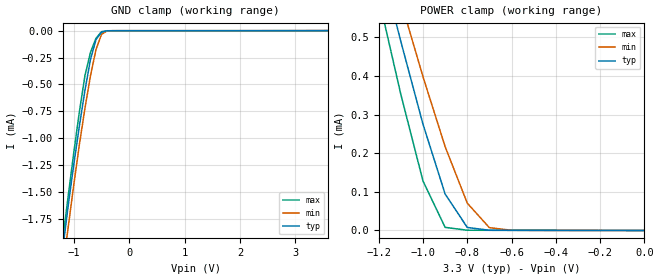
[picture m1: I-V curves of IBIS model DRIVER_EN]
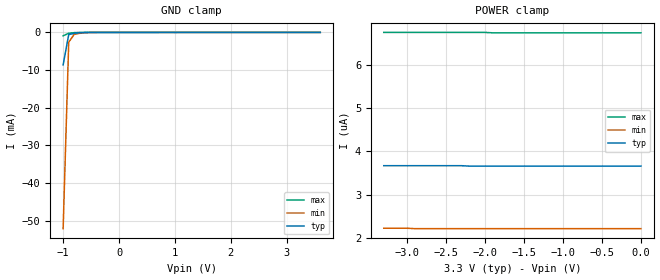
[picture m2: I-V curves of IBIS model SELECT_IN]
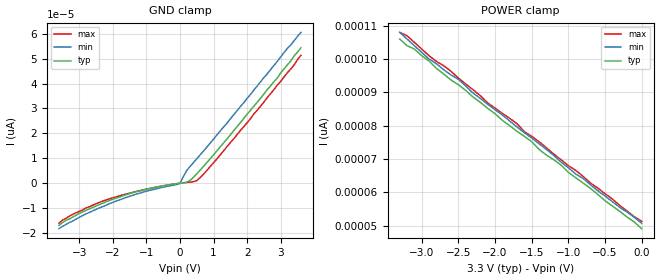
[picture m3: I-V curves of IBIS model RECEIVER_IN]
|   Texas Instruments Incorporated
|   Data Transmissions Products
|   IBIS Model for SN65LVDS125A
|   38DBT TSSOP Package
[IBIS Ver]   3.2
[Comment char]   |_char
[File name]   lvds125a.ibs
[File Rev]   2.1
[Date]   28Jan04
[Source]   File originated at Texas Instruments Incorporated.
   Data Transmission Products Group. All data based on
   Simulation Measurements.
[Notes]   Correlated to Silicon.
[Disclaimer]
(C) Copyright Texas Instruments Incorporated 2004
   All rights reserved
  Texas Instruments Incorporated hereby grants the user of this IBIS
model a non-exclusive, nontransferable license to use this IBIS model
under the following terms.  Before using this IBIS model, the user
should read this license.  If the user does not accept these terms,
the IBIS model should be returned to Texas Instruments within 30 days.
  The user is granted this license only to use the IBIS model and
is not granted rights to sell, load, rent, lease or license the IBIS
model in whole or in part, or in modified form to anyone other than
user.  User may modify the IBIS model to suit its specific applications
but rights to derivative works and such modifications shall belong to
Texas Instruments.
  This IBIS model is provided on an "AS IS" basis and Texas Instruments
makes absolutely no warranty with respect to the information contained
herein.  TEXAS INSTRUMENTS DISCLAIMS AND CUSTOMER WAIVES ALL WARRANTIES,
EXPRESS OR IMPLIED, INCLUDING WARRANTIES OF MERCHANTABILITY OR FITNESS
FOR A PARTICULAR PURPOSE. The entire risk as to quality and performance
is with the Customer. ACCORDINGLY, IN NO EVENT SHALL THE COMPANY BE LIABLE
FOR ANY DAMAGES, WHETHER IN CONTRACT OR TORT,INCLUDING ANY LOST PROFITS
OR OTHER INCIDENTAL, CONSEQUENTIAL, EXEMPLARY, OR PUNITIVE DAMAGES ARISING
OUT OF THE USE OR APPLICATION OF THE IBIS model provided in this package.
Further, Texas Instruments reserves the right to discontinue or make changes
without notice to any product herein to improve reliability, function, or
design. Texas Instruments does not convey any license under patent rights
or any other intellectual property rights, including those of third parties.
Contact Texas Instruments at ATTN:DATA TRANSMISSIONS
[Copyright]   Copyright 2004, Texas Instruments, All Rights Reserved
[Component]   SN65LVDS125A
[Manufacturer]  Texas Instruments Incorporated
[Package]
|   typ   min   max
R_pkg   0.045   0.036   0.057
L_pkg   2.694nH   2.290nH   3.177nH
C_pkg   0.156pF   0.076pF   0.259pF
[Pin]   signal_name   model_name   R_pin   L_pin   C_pin
1   S10   SELECT_IN   0.036   3.045nH   0.259pF
2   S11   SELECT_IN   0.051   3.013nH   0.189pF
3   1A   RECEIVER_IN   0.044   2.695nH   0.164pF
4   1B   RECEIVER_IN   0.047   2.362nH   0.079pF
5   S20   SELECT_IN   0.047   2.333nH   0.086pF
6   S21   SELECT_IN   0.047   2.298nH   0.085pF
7   2A   RECEIVER_IN   0.047   2.351nH   0.079pF
8   2B   RECEIVER_IN   0.044   2.706nH   0.165pF
9   GND   GND   0.049   2.999nH   0.188pF
10   VCC   POWER   0.039   3.039nH   0.257pF
11   GND   GND   0.038   3.044nH   0.258pF
12   3A   RECEIVER_IN   0.057   3.177nH   0.199pF
13   3B   RECEIVER_IN   0.044   2.825nH   0.173pF
14   S30   SELECT_IN   0.047   2.429nH   0.083pF
15   S31   SELECT_IN   0.049   2.383nH   0.090pF
16   4A   RECEIVER_IN   0.049   2.347nH   0.089pF
17   4B   RECEIVER_IN   0.047   2.290nH   0.076pF
18   S40   SELECT_IN   0.045   2.613nH   0.158pF
19   S41   SELECT_IN   0.044   2.883nH   0.181pF
20   VCC   POWER   0.039   3.044nH   0.256pF
21   GND   GND   0.038   3.044nH   0.258pF
22   4DE   DRIVER_EN   0.044   2.883nH   0.181pF
23   4Z   DRIVER_OUT   0.044   2.883nH   0.181pF
24   4Y   DRIVER_OUT   0.044   2.883nH   0.181pF
25   3DE   DRIVER_EN   0.044   2.883nH   0.181pF
26   3Z   DRIVER_OUT   0.044   2.883nH   0.181pF
27   3Y   DRIVER_OUT   0.044   2.883nH   0.181pF
28   GND   GND   0.049   2.999nH   0.188pF
29   VCC   POWER   0.039   3.039nH   0.257pF
30   GND   GND   0.038   3.044nH   0.258pF
31   2DE   DRIVER_EN   0.044   2.883nH   0.181pF
32   2Z   DRIVER_OUT   0.044   2.883nH   0.181pF
33   2Y   DRIVER_OUT   0.044   2.883nH   0.181pF
34   1DE   DRIVER_EN   0.044   2.883nH   0.181pF
35   1Z   DRIVER_OUT   0.044   2.883nH   0.181pF
36   1Y   DRIVER_OUT   0.044   2.883nH   0.181pF
37   GND   GND   0.049   2.999nH   0.188pF
38   VCC   POWER   0.039   3.039nH   0.257pF
[Diff_pin]   inv_pin   vdiff   tdelay_typ   tdelay_min   tdelay_max
| The 'A' or 'Y' pins are Diff_pins and the 'B' or 'Z' pins are inv_pins
   3   4   50m   0   0   0
   7   8   50m   0   0   0
   12   13   50m   0   0   0
   16   17   50m   0   0   0
   24   23   NA   0   0   0
   27   26   NA   0   0   0
   33   32   NA   0   0   0
   36   35   NA   0   0   0
| Models and submodels in the file (4): DRIVER_EN (Input), SELECT_IN (Input), RECEIVER_IN (Input), DRIVER_OUT (3-state)
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|   Driver/Driver Enable Model
[Model]   DRIVER_EN
Model_type   Input
|Signals   1DE,2DE,3DE,4DE
Vinh = 2.0
Vinl = 0.8
|   typ   min   max
C_comp   2.72pF   2.57pF   2.79pF
|   typ   min   max
[Temperature Range]   25.0   85.0   -40.0
[Voltage range]   3.3V   3.0V   3.6V
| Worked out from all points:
|   GND clamp passes 1 mA (typ) near -0.93 V on its own axis
|   POWER clamp passes 1 mA (typ) near -1.32 V on its own axis
[GND_clamp]
|   Voltage   I(typ)   I(min)   I(max)
-3.6V     -14.2mA    -13.5mA    -15mA
-1.2V     -2.03mA    -2.22mA    -1.94mA
-1.1V     -1.62mA    -1.82mA    -1.53mA
-1V       -1.24mA    -1.43mA    -1.13mA
-900mV    -887uA     -1.06mA    -754uA
-800mV    -557uA     -724uA     -420uA
-700mV    -269uA     -421uA     -203uA
-600mV    -83.9uA    -176uA     -71.3uA
-500mV    -14.8uA    -34.1uA    -9.02uA
-400mV    -1.52uA    -3.27uA    -1.07uA
-300mV    -611nA     -591nA     -834nA
3.6V      162nA      572nA      40.6pA
[Power_clamp]
| Note that the[POWER_clamp]voltage table is referenced to Vcc
| and is calculated using Vtable=Vcc - Vmeasured.
|   Voltage   I(typ)   I(min)   I(max)
-3.3V     5.83mA     5.35mA     6.36mA
-1.2V     714uA      796uA      602uA
-1.1V     489uA      593uA      352uA
-1V       275uA      398uA      128uA
-900mV    94.4uA     217uA      8.05uA
-800mV    7.83uA     70.7uA     648nA
-700mV    564nA      7.24uA     514nA
-600mV    340nA      572nA      438nA
0V        43.3pA     123pA      40.6pA
|   Select Pin Model
[Model]   SELECT_IN
Model_type   Input
|Signals   S10,S11,S20,S21,S30,S31,S40,S41
Vinh = 2.0
Vinl = 0.8
|   typ   min   max
C_comp   3.31pF   3.28pF   3.38pF
|   typ   min   max
[Temperature Range]   25.0   85   -40
[Voltage range]   3.3V   3.0V   3.6V
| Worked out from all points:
|   GND clamp passes 1 mA (typ) near -0.91 V on its own axis
[GND_clamp]
|   Voltage   I(typ)   I(min)   I(max)
-1V       -8.62mA    -52.1mA    -903uA
-900mV    -570uA     -2.59mA    -220uA
-800mV    -233uA     -479uA     -60.3uA
-400mV    -1.44uA    -1.66uA    -2.45uA
3.6V      3.66uA     2.22uA     6.73uA
[Power_clamp]
| Note that the[POWER_clamp]voltage table is referenced to Vcc
| and is calculated using Vtable=Vcc - Vmeasured.
|   Voltage   I(typ)   I(min)   I(max)
-3.3V     3.67uA     2.23uA     6.74uA
-3V       3.67uA     2.23uA     6.74uA
-2.9V     3.67uA     2.22uA     6.74uA
-2.3V     3.67uA     2.22uA     6.74uA
-2.2V     3.66uA     2.22uA     6.74uA
-2V       3.66uA     2.22uA     6.74uA
-1.9V     3.66uA     2.22uA     6.73uA
0V        3.66uA     2.22uA     6.73uA
|   Receiver Input Model
[Model]   RECEIVER_IN
Model_type   Input
|Signals   1A,1B,2A,2B,3A,3B,4A,4B
Vinh = 1.4
Vinl = 1.0
|   typ   min   max
C_comp   2.58pF   2.47pF   2.64pF
|   typ   min   max
[Temperature Range]   25.0   85   -40
[Voltage range]   3.3V   3.0V   3.6V
[GND_clamp]
|   Voltage   I(typ)   I(min)   I(max)
-3.6V     -16.9pA    -18.2pA    -16pA
-3.2V     -13.6pA    -15.2pA    -12.5pA
-2.1V     -6.89pA    -8.18pA    -6.24pA
-1.2V     -3.03pA    -3.96pA    -3.01pA
0V        0A         0A         0A
200mV     412fA      5.09pA     319fA
500mV     3.77pA     9.79pA     1.06pA
1V        11.4pA     17.7pA     8.23pA
2.1V      29.3pA     35.6pA     25.9pA
2.9V      42.2pA     48.9pA     39.4pA
3.3V      49.1pA     55.5pA     45.8pA
3.6V      54.3pA     60.5pA     51.3pA
[Power_clamp]
| Note that the[POWER_clamp]voltage table is referenced to Vcc
| and is calculated using Vtable=Vcc - Vmeasured.
|   Voltage   I(typ)   I(min)   I(max)
-3.3V     106pA      108pA      108pA
-3.2V     104pA      106pA      107pA
-3.1V     103pA      104pA      105pA
-2.9V     99.4pA     100pA      101pA
-2.8V     97.2pA     98.6pA     99.3pA
-2.5V     92.3pA     93.9pA     94.3pA
-2.1V     85.2pA     86.4pA     86.8pA
-1.7V     78.3pA     79.6pA     80.6pA
-1.6V     76.8pA     77.9pA     78.2pA
-900mV    64.4pA     65.5pA     66.6pA
-700mV    61.2pA     62.3pA     62.8pA
0V        49.1pA     50.7pA     51.3pA
